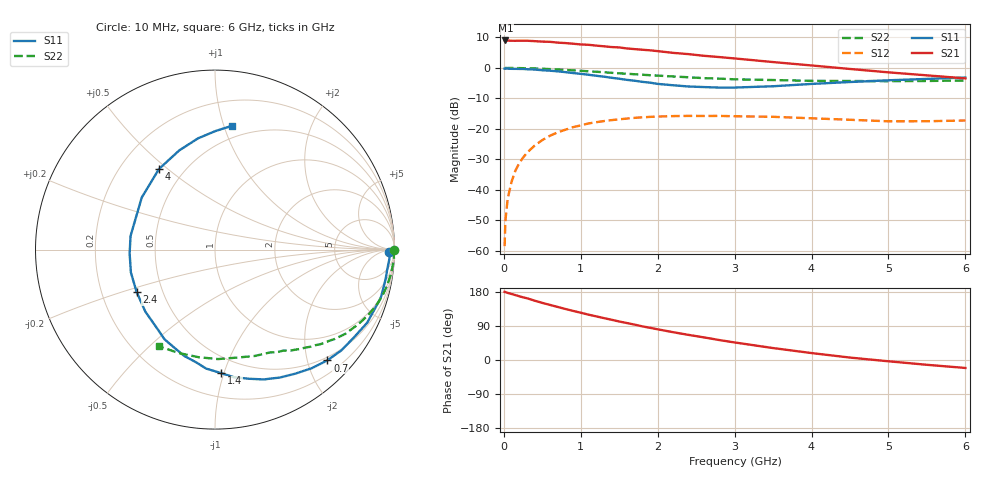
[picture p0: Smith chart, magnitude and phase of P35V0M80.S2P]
! SIEMENS Small Signal Semiconductors
! BFP181
! Si NPN RF Bipolar Junction Transistor in SOT143
! VCE = 5 V  IC = 0.8 mA
! Common Emitter S-Parameters:  March  1996
# GHz  S  MA  R  50
!  f  S11  S21  S12  S22
! GHz  MAG  ANG  MAG  ANG  MAG  ANG  MAG  ANG
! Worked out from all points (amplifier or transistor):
!   36 points, 10 MHz to 6 GHz, reference 50 ohm
!   highest |S21| = 9.0 dB at 20 MHz (marker M1)
!   |S21| within 3 dB of that: start of sweep to 1.78 GHz
!   unconditionally stable (mu >= 1): 3.424 GHz to end of sweep
!   at 250 MHz: K = 0.09, MSG = 19.1 dB, |S12| = -29.4 dB
!   at 1.4 GHz: K = 0.46, MSG = 12.0 dB, |S12| = -17.1 dB
!   at 6 GHz: K = 1.33, MAG = 3.5 dB, |S12| = -17.2 dB
!   S11 on the Smith chart (normalised r, x): 10 MHz: 58, -24; 700 MHz: 0.44, -2.37; 1.4 GHz: 0.37, -0.98; 2.4 GHz: 0.36, -0.22; 4 GHz: 0.36, +0.47; 6 GHz: 0.40, +1.06
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0.01  0.9712 -0.7  2.815 179.7  0.0012 81.7  0.9993 -0.2
0.02  0.9722 -1.2  2.818 179.4  0.0031 88.2  0.9968 -0.6
0.05  0.9733 -3.0  2.804 177.1  0.0072 91.3  0.9963 -1.6
0.1  0.9658 -6.7  2.786 174.3  0.0136 84.7  0.9987 -3.1
0.15  0.9648 -9.6  2.782 171.3  0.0207 82.5  0.9946 -4.6
0.2  0.9624 -12.8  2.794 168.3  0.0275 81.7  0.9927 -6.1
0.3  0.9518 -19.4  2.789 163.0  0.0407 77.0  0.9861 -9.1
0.5  0.9156 -32.3  2.696 150.7  0.0657 68.2  0.9687 -15.0
0.7  0.8791 -44.6  2.598 140.0  0.0879 59.9  0.942 -20.6
0.9  0.8238 -57.0  2.491 129.6  0.107 52.2  0.912 -25.6
1.1  0.7727 -69.4  2.393 119.7  0.1229 45.1  0.8802 -30.3
1.4  0.689 -87.2  2.197 106.2  0.1395 35.7  0.8317 -36.8
1.5  0.6645 -94.3  2.166 101.6  0.1438 33.1  0.8153 -38.5
1.8  0.591 -112.7  1.986 88.8  0.1551 25.8  0.7732 -43.5
2.2  0.5197 -138.3  1.765 73.4  0.1624 16.8  0.7241 -50.0
2.4  0.4964 -151.7  1.683 66.3  0.1636 12.9  0.703 -53.1
3  0.4766 170.8  1.43 46.3  0.1615 3.8  0.6501 -61.8
3.5  0.5007 144.6  1.247 31.5  0.158 -1.7  0.6329 -69.4
4  0.5466 124.9  1.097 18.3  0.1494 -5.3  0.6142 -78.4
4.5  0.5876 109.8  0.961 6.4  0.1413 -7.8  0.6102 -88.5
5.5  0.6605 89.8  0.755 -12.7  0.1337 -3.7  0.6109 -109.5
6  0.6962 82.2  0.674 -21.0  0.1376 -2.0  0.6229 -120.3
